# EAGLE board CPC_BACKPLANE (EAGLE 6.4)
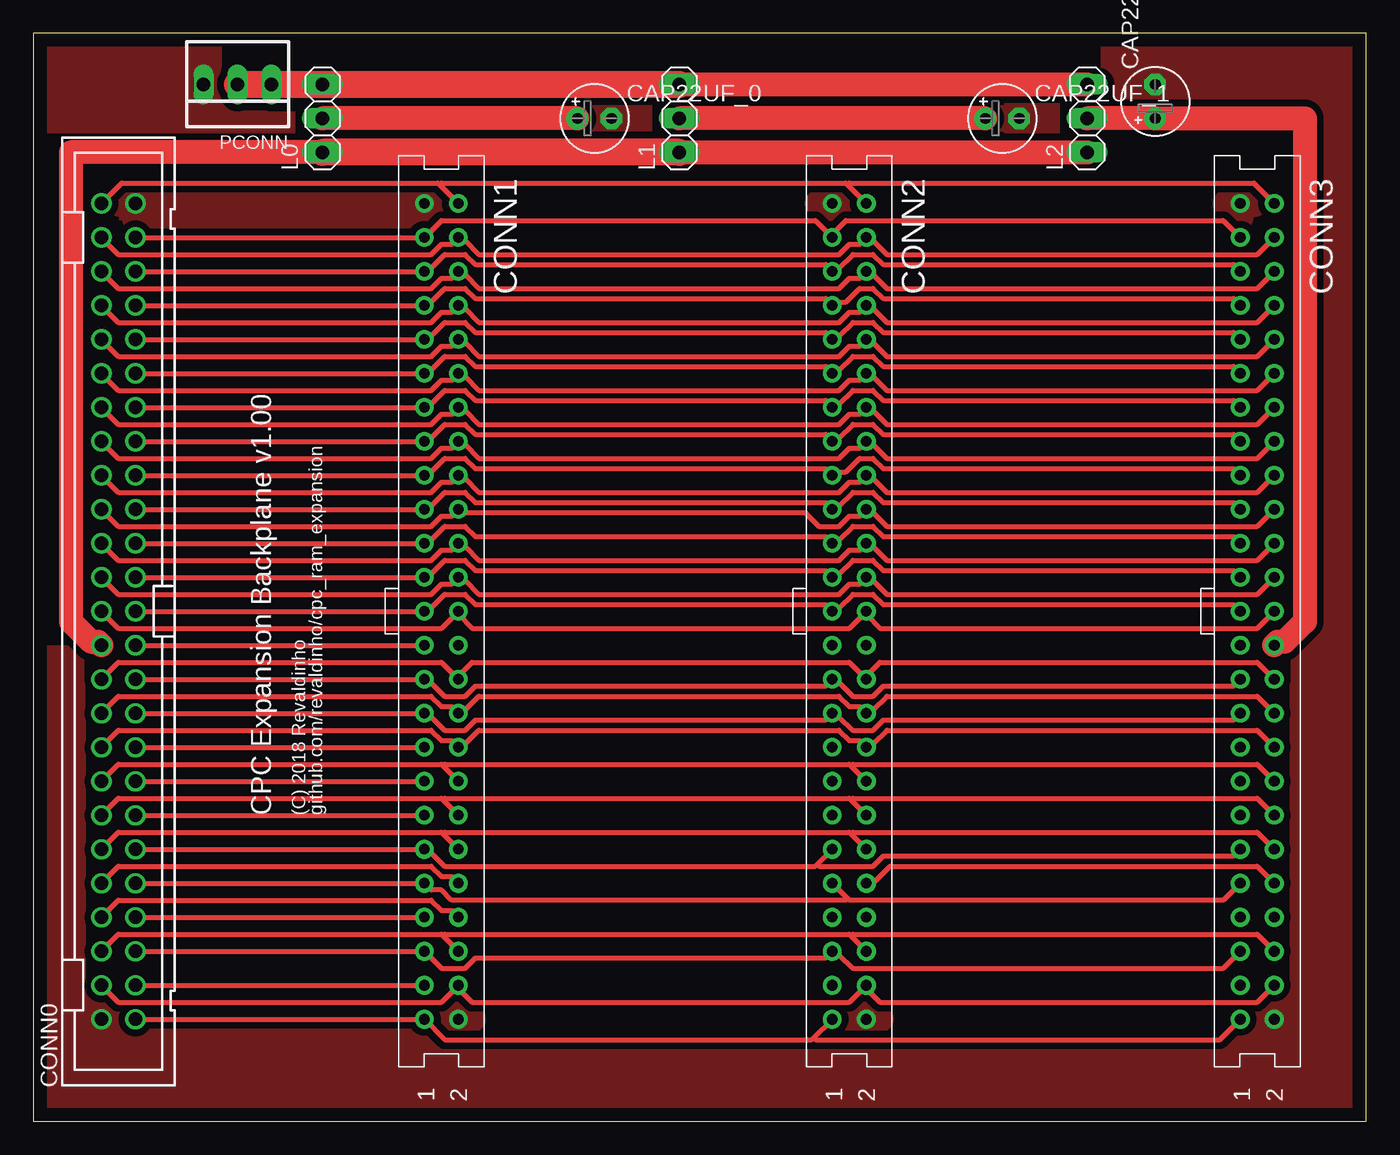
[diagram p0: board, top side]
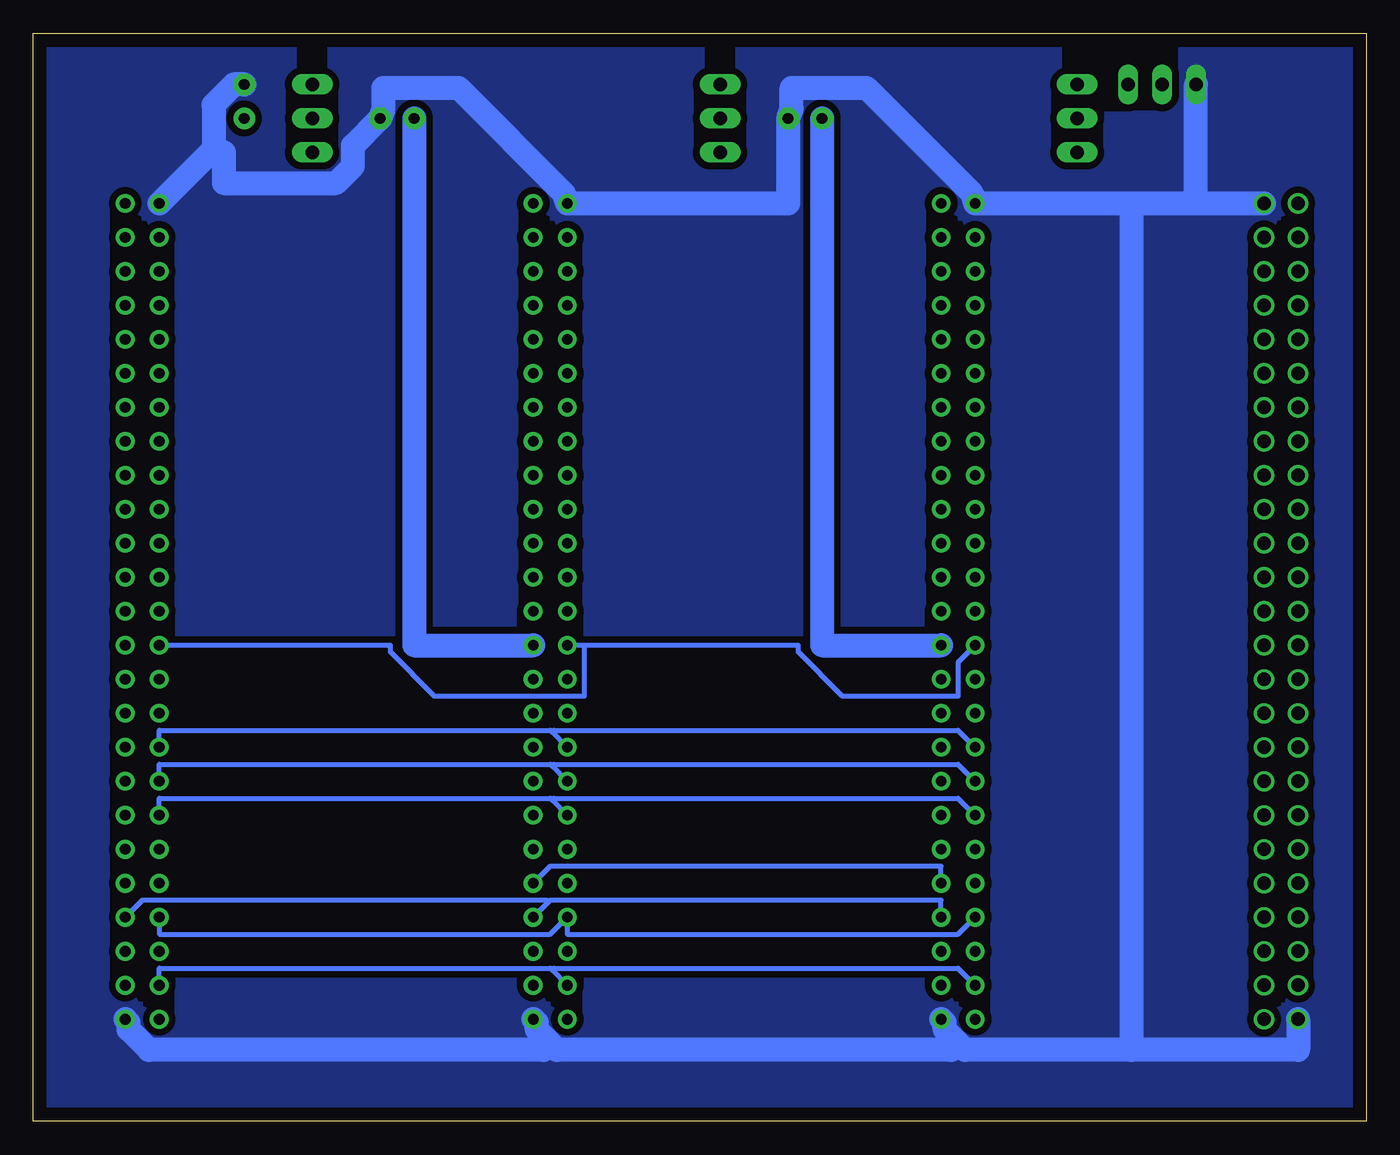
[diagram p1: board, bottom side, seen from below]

Size 99.57 x 81.28 mm. Coordinates in mm from the lower left corner, seen from the top.
Outline: 0,0 99.57,0 99.57,81.28 0,81.28 0,0
Copper layers (1*16): Top 0.035mm / dielectric 1.5mm / Bottom 0.035mm
Design rules "default": minimum track width 10mil, minimum drill 24mil, track to track 8mil, track to pad 8mil, pad to pad 8mil, via to via 8mil, smd to smd 8mil, copper to edge 40mil, drill to drill 8mil, minimum pad ring 10mil, minimum via ring 8mil, stop-mask expansion 4mil, vias tented up to drill 0mil, thermal gap 10mil
Net classes: 0 signal: width 0.381 mm, clearance 0.254 mm; 1 supply: width 1.778 mm, clearance 0.508 mm

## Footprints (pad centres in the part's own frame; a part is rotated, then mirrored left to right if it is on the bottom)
E2,5-5 = drill 0.813 pad 1.6: + -1.27,0 | drill 0.813 pad 1.6 octagon: - 1.27,0
PAK100/2500-50 = drill 1 pad 1.422: 1 -30.48,-1.27; 2 -30.48,1.27; 3 -27.94,-1.27; 4 -27.94,1.27; 5 -25.4,-1.27; 6 -25.4,1.27; 7 -22.86,-1.27; 8 -22.86,1.27; 9 -20.32,-1.27; 10 -20.32,1.27; 11 -17.78,-1.27; 12 -17.78,1.27; 13 -15.24,-1.27; 14 -15.24,1.27; 15 -12.7,-1.27; 16 -12.7,1.27; 17 -10.16,-1.27; 18 -10.16,1.27; 19 -7.62,-1.27; 20 -7.62,1.27; 21 -5.08,-1.27; 22 -5.08,1.27; 23 -2.54,-1.27; 24 -2.54,1.27; 25 0,-1.27; 26 0,1.27; 27 2.54,-1.27; 28 2.54,1.27; 29 5.08,-1.27; 30 5.08,1.27; 31 7.62,-1.27; 32 7.62,1.27; 33 10.16,-1.27; 34 10.16,1.27; 35 12.7,-1.27; 36 12.7,1.27; 37 15.24,-1.27; 38 15.24,1.27; 39 17.78,-1.27; 40 17.78,1.27; 41 20.32,-1.27; 42 20.32,1.27; 43 22.86,-1.27; 44 22.86,1.27; 45 25.4,-1.27; 46 25.4,1.27; 47 27.94,-1.27; 48 27.94,1.27; 49 30.48,-1.27; 50 30.48,1.27
S50V = drill 0.8 pad 1.4: 1 30.48,-1.27; 2 30.48,1.27; 3 27.94,-1.27; 4 27.94,1.27; 5 25.4,-1.27; 6 25.4,1.27; 7 22.86,-1.27; 8 22.86,1.27; 9 20.32,-1.27; 10 20.32,1.27; 11 17.78,-1.27; 12 17.78,1.27; 13 15.24,-1.27; 14 15.24,1.27; 15 12.7,-1.27; 16 12.7,1.27; 17 10.16,-1.27; 18 10.16,1.27; 19 7.62,-1.27; 20 7.62,1.27; 21 5.08,-1.27; 22 5.08,1.27; 23 2.54,-1.27; 24 2.54,1.27; 25 0,-1.27; 26 0,1.27; 27 -2.54,-1.27; 28 -2.54,1.27; 29 -5.08,-1.27; 30 -5.08,1.27; 31 -7.62,-1.27; 32 -7.62,1.27; 33 -10.16,-1.27; 34 -10.16,1.27; 35 -12.7,-1.27; 36 -12.7,1.27; 37 -15.24,-1.27; 38 -15.24,1.27; 39 -17.78,-1.27; 40 -17.78,1.27; 41 -20.32,-1.27; 42 -20.32,1.27; 43 -22.86,-1.27; 44 -22.86,1.27; 45 -25.4,-1.27; 46 -25.4,1.27; 47 -27.94,-1.27; 48 -27.94,1.27; 49 -30.48,-1.27; 50 -30.48,1.27
1X03 = drill 1.016 long: 1 -2.54,0; 2 0,0; 3 2.54,0
22-23-2031 = drill 1 long: 1 -2.54,0; 2 0,0; 3 2.54,0

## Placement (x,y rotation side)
CAP22UF_0  [E2,5-5]  41.91,74.93 0 top
CAP22UF_1  [E2,5-5]  72.39,74.93 0 top
CAP22UF_2  [E2,5-5]  83.82,76.2 90 top
CONN0  [PAK100/2500-50]  6.35,38.1 90 top
CONN1  [S50V]  30.48,38.1 270 top
CONN2  [S50V]  60.96,38.1 270 top
CONN3  [S50V]  91.44,38.1 270 top
L0  [1X03]  21.59,74.93 90 top
L1  [1X03]  48.26,74.93 90 top
L2  [1X03]  78.74,74.93 90 top
PCONN  [22-23-2031]  15.24,77.47 180 top

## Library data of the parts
CAP22UF_0 CAP22UF_1 CAP22UF_2 = resistor
CONN0 = con-3m
CONN1-CONN3 = con-3m-skt-header
L0 L1 L2 = pinhead
PCONN = con-molex

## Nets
A0: CONN0.33 CONN1.33 CONN2.33 CONN3.33
A1: CONN0.34 CONN1.34 CONN2.34 CONN3.34
A2: CONN0.35 CONN1.35 CONN2.35 CONN3.35
A3: CONN0.36 CONN1.36 CONN2.36 CONN3.36
A4: CONN0.37 CONN1.37 CONN2.37 CONN3.37
A5: CONN0.38 CONN1.38 CONN2.38 CONN3.38
A6: CONN0.39 CONN1.39 CONN2.39 CONN3.39
A7: CONN0.40 CONN1.40 CONN2.40 CONN3.40
A8: CONN0.41 CONN1.41 CONN2.41 CONN3.41
A9: CONN0.42 CONN1.42 CONN2.42 CONN3.42
A10: CONN0.43 CONN1.43 CONN2.43 CONN3.43
A11: CONN0.44 CONN1.44 CONN2.44 CONN3.44
A12: CONN0.45 CONN1.45 CONN2.45 CONN3.45
A13: CONN0.46 CONN1.46 CONN2.46 CONN3.46
A14: CONN0.47 CONN1.47 CONN2.47 CONN3.47
A15: CONN0.48 CONN1.48 CONN2.48 CONN3.48
BUSACK_B: CONN0.13 CONN1.13 CONN2.13 CONN3.13
BUSRESET_B: CONN0.11 CONN1.11 CONN2.11 CONN3.11
BUSRQ_B: CONN0.14 CONN1.14 CONN2.14 CONN3.14
CLK: CONN0.1 CONN1.1 CONN2.1 CONN3.1
CURSOR: CONN0.5 CONN1.5 CONN2.5 CONN3.5
D0: CONN0.25 CONN1.25 CONN2.25 CONN3.25
D1: CONN0.26 CONN1.26 CONN2.26 CONN3.26
D2: CONN0.27 CONN1.27 CONN2.27 CONN3.27
D3: CONN0.28 CONN1.28 CONN2.28 CONN3.28
D4: CONN0.29 CONN1.29 CONN2.29 CONN3.29
D5: CONN0.30 CONN1.30 CONN2.30 CONN3.30
D6: CONN0.31 CONN1.31 CONN2.31 CONN3.31
D7: CONN0.32 CONN1.32 CONN2.32 CONN3.32
EXP_B: CONN0.3 CONN1.3 CONN2.3 CONN3.3
HALT_B: CONN0.17 CONN1.17 CONN2.17 CONN3.17
INT_B: CONN0.16 CONN1.16 CONN2.16 CONN3.16
IOREQ_B: CONN0.20 CONN1.20 CONN2.20 CONN3.20
LPEN: CONN0.4 CONN1.4 CONN2.4 CONN3.4
M1_B: CONN0.22 CONN1.22 CONN2.22 CONN3.22
MREQ_B: CONN0.23 CONN1.23 CONN2.23 CONN3.23
NMI_B: CONN0.15 CONN1.15 CONN2.15 CONN3.15
RAMDIS: CONN0.6 CONN1.6 CONN2.6 CONN3.6
RAMRD_B: CONN0.7 CONN1.7 CONN2.7 CONN3.7
RD_B: CONN0.19 CONN1.19 CONN2.19 CONN3.19
READY: CONN0.12 CONN1.12 CONN2.12 CONN3.12
RESET_B: CONN0.10 CONN1.10 CONN2.10 CONN3.10
RFSH_B: CONN0.21 CONN1.21 CONN2.21 CONN3.21
ROMDIS: CONN0.8 CONN1.8 CONN2.8 CONN3.8
ROMEN_B: CONN0.9 CONN1.9 CONN2.9 CONN3.9
SOUND: CONN0.50 CONN1.50 CONN2.50 CONN3.50
VDD [supply]: CAP22UF_0.+ CONN1.24 L0.2
VDD2 [supply]: CAP22UF_1.+ CONN2.24 L1.2
VDD3 [supply]: CAP22UF_2.+ CONN3.24 L2.2
VDD_CPC [supply]: CONN0.24 L0.1 L1.1 L2.1
VDD_EXT [supply]: L0.3 L1.3 L2.3 PCONN.1 PCONN.2
VSS [supply]: CAP22UF_0.- CAP22UF_1.- CAP22UF_2.- CONN0.2 CONN0.49 CONN1.2 CONN1.49 CONN2.2 CONN2.49 CONN3.2 CONN3.49 PCONN.3
WR_B: CONN0.18 CONN1.18 CONN2.18 CONN3.18

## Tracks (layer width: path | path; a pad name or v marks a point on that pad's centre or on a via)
A0
  Top 0.381: CONN0.33 CONN1.33 29.46,48.26 30.73,49.53 32.26,49.53 33.02,48.77 59.18,48.77 CONN2.33 59.69,48.51 60.71,48.51 61.72,49.53 62.74,49.53 63.5,48.77 89.66,48.77 CONN3.33
A1
  Top 0.381: CONN0.34 6.35,46.99 29.72,46.99 30.48,47.75 31.24,47.75 CONN1.34 31.75,48.01 32.26,48.01 33.27,46.99 60.2,46.99 60.96,47.75 61.72,47.75 CONN2.34 62.23,48.01 62.74,48.01 63.75,46.99 91.44,46.99 CONN3.34
A2
  Top 0.381: CONN0.35 CONN1.35 29.46,50.8 30.73,52.07 32.26,52.07 33.02,51.31 59.18,51.31 CONN2.35 59.69,51.05 60.2,51.05 61.21,52.07 62.74,52.07 63.5,51.31 89.66,51.31 CONN3.35
A3
  Top 0.381: CONN0.36 6.35,49.53 29.72,49.53 30.48,50.29 31.24,50.29 CONN1.36 31.75,50.55 32.26,50.55 33.27,49.53 60.2,49.53 60.96,50.29 61.72,50.29 CONN2.36 62.23,50.55 62.74,50.55 63.75,49.53 91.44,49.53 CONN3.36
A4
  Top 0.381: CONN0.37 CONN1.37 29.46,53.34 30.73,54.61 32.26,54.61 33.02,53.85 59.18,53.85 CONN2.37 59.69,53.59 60.2,53.59 61.21,54.61 62.74,54.61 63.5,53.85 89.66,53.85 CONN3.37
A5
  Top 0.381: CONN0.38 6.35,52.07 29.72,52.07 30.48,52.83 31.24,52.83 CONN1.38 31.75,53.09 32.26,53.09 33.27,52.07 60.2,52.07 60.96,52.83 61.72,52.83 CONN2.38 62.23,53.09 62.74,53.09 63.75,52.07 91.44,52.07 CONN3.38
A6
  Top 0.381: CONN0.39 CONN1.39 29.46,55.88 30.73,57.15 32.26,57.15 33.02,56.39 59.18,56.39 CONN2.39 59.69,56.13 60.2,56.13 61.21,57.15 62.74,57.15 63.5,56.39 89.66,56.39 CONN3.39
A7
  Top 0.381: CONN0.40 6.35,54.61 29.72,54.61 30.48,55.37 31.24,55.37 CONN1.40 31.75,55.63 32.26,55.63 33.27,54.61 60.2,54.61 60.96,55.37 61.72,55.37 CONN2.40 62.23,55.63 62.74,55.63 63.75,54.61 91.44,54.61 CONN3.40
A8
  Top 0.381: CONN0.41 CONN1.41 29.46,58.42 30.73,59.69 32.26,59.69 33.02,58.93 59.18,58.93 CONN2.41 59.69,58.67 60.2,58.67 61.21,59.69 62.74,59.69 63.5,58.93 89.66,58.93 CONN3.41
A9
  Top 0.381: CONN0.42 6.35,57.15 29.72,57.15 30.48,57.91 31.24,57.91 CONN1.42 31.75,58.17 32.26,58.17 33.27,57.15 60.2,57.15 60.96,57.91 61.72,57.91 CONN2.42 62.23,58.17 62.74,58.17 63.75,57.15 91.44,57.15 CONN3.42
A10
  Top 0.381: CONN0.43 CONN1.43 29.46,60.96 30.73,62.23 32.26,62.23 33.02,61.47 59.18,61.47 CONN2.43 59.69,61.21 60.71,61.21 61.72,62.23 62.74,62.23 63.5,61.47 89.66,61.47 CONN3.43
A11
  Top 0.381: CONN0.44 6.35,59.69 29.72,59.69 30.48,60.45 31.24,60.45 CONN1.44 31.75,60.71 32.26,60.71 33.27,59.69 60.2,59.69 60.96,60.45 61.72,60.45 CONN2.44 62.23,60.71 62.74,60.71 63.75,59.69 91.44,59.69 CONN3.44
A12
  Top 0.381: CONN0.45 CONN1.45 29.46,63.5 30.73,64.77 32.26,64.77 33.02,64.01 59.18,64.01 CONN2.45 59.69,63.75 60.2,63.75 61.21,64.77 62.74,64.77 63.5,64.01 89.66,64.01 CONN3.45
A13
  Top 0.381: CONN0.46 6.35,62.23 29.72,62.23 30.48,62.99 31.24,62.99 CONN1.46 31.75,63.25 32.26,63.25 33.27,62.23 60.2,62.23 60.96,62.99 61.72,62.99 CONN2.46 62.23,63.25 62.74,63.25 63.75,62.23 91.44,62.23 CONN3.46
A14
  Top 0.381: CONN0.47 CONN1.47 30.48,67.31 58.42,67.31 CONN2.47 59.69,66.29 60.71,67.31 88.9,67.31 CONN3.47
A15
  Top 0.381: CONN0.48 6.35,64.77 29.72,64.77 30.48,65.53 31.24,65.53 CONN1.48 31.75,65.79 32.26,65.79 33.27,64.77 60.2,64.77 60.96,65.53 61.72,65.53 CONN2.48 62.23,65.79 62.74,65.79 63.75,64.77 91.44,64.77 CONN3.48
BUSACK_B
  Top 0.381: CONN0.13 CONN1.13
  Bottom 0.381: 60.83,24 60.96,24.13 90.17,24.13 CONN3.13 | 60.83,24 CONN2.13 | CONN1.13 30.48,24.13 60.71,24.13 60.83,24
BUSRESET_B
  Top 0.381: CONN0.11 CONN1.11 29.46,20.32 30.73,19.05 58.42,19.05 58.55,19.18 | 58.55,19.18 CONN2.11 | CONN3.11 89.66,19.81 63.5,19.81 62.74,19.05 58.67,19.05 58.55,19.18
BUSRQ_B
  Top 0.381: 30.61,24 30.48,24.13 6.35,24.13 CONN0.14 | 30.61,24 CONN1.14 | 61.09,24 60.96,24.13 30.73,24.13 30.61,24 | 61.09,24 CONN2.14 | CONN3.14 91.44,24.13 61.21,24.13 61.09,24
CLK
  Top 0.381: CONN0.1 CONN1.1 30.73,6.1 58.17,6.1 58.29,6.22 | 58.29,6.22 CONN2.1 | CONN3.1 88.65,6.1 58.42,6.1 58.29,6.22
CURSOR
  Top 0.381: CONN0.5 CONN1.5 30.48,11.43 32.26,11.43 33.02,12.19 59.18,12.19 CONN2.5 59.69,12.45 60.2,12.45 61.21,11.43 88.9,11.43 CONN3.5
D0
  Top 0.381: CONN0.25 CONN1.25 29.46,38.1 30.73,39.37 32.26,39.37 33.02,38.61 59.18,38.61 CONN2.25 59.69,38.35 60.2,38.35 61.21,39.37 62.74,39.37 63.5,38.61 89.66,38.61 CONN3.25
D1
  Top 0.381: CONN0.26 6.35,36.83 30.48,36.83 CONN1.26 31.75,37.85 32.77,36.83 60.96,36.83 CONN2.26 62.23,37.85 63.25,36.83 91.44,36.83 CONN3.26
D2
  Top 0.381: CONN0.27 CONN1.27 29.46,40.64 30.73,41.91 32.26,41.91 33.02,41.15 59.18,41.15 CONN2.27 59.69,40.89 60.2,40.89 61.21,41.91 62.74,41.91 63.5,41.15 89.66,41.15 CONN3.27
D3
  Top 0.381: CONN0.28 6.35,39.37 29.72,39.37 30.48,40.13 31.24,40.13 CONN1.28 31.75,40.39 32.26,40.39 33.27,39.37 60.2,39.37 60.96,40.13 61.72,40.13 CONN2.28 62.23,40.39 62.74,40.39 63.75,39.37 91.44,39.37 CONN3.28
D4
  Top 0.381: CONN0.29 CONN1.29 29.46,43.18 30.73,44.45 32.26,44.45 33.02,43.69 59.18,43.69 CONN2.29 59.69,43.43 60.2,43.43 61.21,44.45 62.74,44.45 63.5,43.69 89.66,43.69 CONN3.29
D5
  Top 0.381: CONN0.30 6.35,41.91 29.72,41.91 30.48,42.67 31.24,42.67 CONN1.30 31.75,42.93 32.26,42.93 33.27,41.91 60.2,41.91 60.96,42.67 61.72,42.67 CONN2.30 62.23,42.93 62.74,42.93 63.75,41.91 91.44,41.91 CONN3.30
D6
  Top 0.381: CONN0.31 CONN1.31 29.46,45.72 30.73,46.99 32.26,46.99 33.02,46.23 59.18,46.23 CONN2.31 59.69,45.97 60.2,45.97 61.21,46.99 62.74,46.99 63.5,46.23 89.66,46.23 CONN3.31
D7
  Top 0.381: CONN0.32 6.35,44.45 29.72,44.45 30.48,45.21 31.24,45.21 CONN1.32 31.75,45.47 57.66,45.47 58.67,44.45 60.2,44.45 60.96,45.21 61.72,45.21 CONN2.32 62.23,45.47 62.74,45.47 63.75,44.45 91.44,44.45 CONN3.32
EXP_B
  Top 0.381: CONN0.3 CONN1.3
  Bottom 0.381: 60.83,11.3 60.96,11.43 90.17,11.43 CONN3.3 | 60.83,11.3 CONN2.3 | CONN1.3 30.48,11.43 60.71,11.43 60.83,11.3
HALT_B
  Top 0.381: CONN0.17 CONN1.17
  Bottom 0.381: 60.83,29.08 60.96,29.21 90.17,29.21 CONN3.17 | 60.83,29.08 CONN2.17 | CONN1.17 30.48,29.21 60.71,29.21 60.83,29.08
INT_B
  Top 0.381: 30.61,26.54 30.48,26.67 6.35,26.67 CONN0.16 | 30.61,26.54 CONN1.16 | 61.09,26.54 60.96,26.67 30.73,26.67 30.61,26.54 | 61.09,26.54 CONN2.16 | CONN3.16 91.44,26.67 61.21,26.67 61.09,26.54
IOREQ_B
  Top 0.381: CONN0.20 6.35,31.75 29.72,31.75 30.48,30.99 31.24,30.99 CONN1.20 31.75,30.73 32.26,30.73 33.27,31.75 60.2,31.75 60.96,30.99 61.72,30.99 CONN2.20 62.23,30.73 62.74,30.73 63.75,31.75 91.44,31.75 CONN3.20
LPEN
  Top 0.381: CONN0.4 6.35,8.89 30.48,8.89 CONN1.4 31.75,9.91 32.77,8.89 60.96,8.89 CONN2.4 62.23,9.91 63.25,8.89 91.44,8.89 CONN3.4
M1_B
  Top 0.381: CONN0.22 6.35,34.29 30.48,34.29 CONN1.22 31.75,33.27 32.77,34.29 60.96,34.29 CONN2.22 62.23,33.27 63.25,34.29 91.44,34.29 CONN3.22
MREQ_B
  Top 0.381: CONN0.23 CONN1.23
  Bottom 0.381: 58.42,35.56 42.42,35.56 42.42,35.05 39.12,31.75 30.48,31.75 30.48,34.29 CONN1.23 | 58.42,35.56 CONN2.23 | CONN3.23 72.9,35.56 72.9,35.05 69.6,31.75 58.42,31.75 58.42,35.56
NMI_B
  Top 0.381: CONN0.15 CONN1.15
  Bottom 0.381: 60.83,26.54 60.96,26.67 90.17,26.67 CONN3.15 | 60.83,26.54 CONN2.15 | CONN1.15 30.48,26.67 60.71,26.67 60.83,26.54
RAMDIS
  Top 0.381: 30.61,13.84 30.48,13.97 6.35,13.97 CONN0.6 | 30.61,13.84 CONN1.6 | 61.09,13.84 60.96,13.97 30.73,13.97 30.61,13.84 | 61.09,13.84 CONN2.6 | CONN3.6 91.44,13.97 61.21,13.97 61.09,13.84
RAMRD_B
  Top 0.381: CONN0.7 CONN1.7
  Bottom 0.381: CONN3.7 90.17,13.97 60.96,13.97 CONN2.7 59.69,13.97 30.48,13.97 CONN1.7
RD_B
  Top 0.381: CONN0.19 CONN1.19 29.46,30.48 30.73,29.21 32.26,29.21 33.02,29.97 59.18,29.97 CONN2.19 59.69,30.23 60.2,30.23 61.21,29.21 62.74,29.21 63.5,29.97 89.66,29.97 CONN3.19
READY
  Top 0.381: 30.61,21.46 30.48,21.59 6.35,21.59 CONN0.12 | 30.61,21.46 CONN1.12 | 61.09,21.46 60.96,21.59 30.73,21.59 30.61,21.46 | 61.09,21.46 CONN2.12 | CONN3.12 91.44,21.59 61.21,21.59 61.09,21.46
RESET_B
  Top 0.381: CONN1.10 31.24,18.29 30.48,18.29 29.72,19.05 6.35,19.05 CONN0.10 | CONN3.10 91.44,19.05 64.01,19.05 62.74,17.78 CONN2.10
  Bottom 0.381: CONN2.10 60.96,19.05 31.75,19.05 CONN1.10
RFSH_B
  Top 0.381: CONN0.21 CONN1.21 29.46,33.02 30.73,31.75 32.26,31.75 33.02,32.51 59.18,32.51 CONN2.21 59.69,32.77 60.2,32.77 61.21,31.75 62.74,31.75 63.5,32.51 89.66,32.51 CONN3.21
ROMDIS
  Top 0.381: CONN1.8 31.24,15.75 30.48,15.75 29.72,16.51 6.35,16.51 CONN0.8
  Bottom 0.381: 61.09,16.38 60.96,16.51 31.75,16.51 CONN1.8 | 61.09,16.38 CONN2.8 | CONN3.8 91.44,16.51 61.21,16.51 61.09,16.38
ROMEN_B
  Top 0.381: CONN0.9 CONN1.9 29.72,17.27 30.48,17.27 31.24,16.51 60.71,16.51 60.83,16.64 | 60.83,16.64 60.96,16.51 88.9,16.51 CONN3.9 | 60.83,16.64 CONN2.9
SOUND
  Top 0.381: 30.35,69.98 30.23,70.1 6.6,70.1 CONN0.50 | 30.35,69.98 CONN1.50 | 60.83,69.98 60.71,70.1 30.48,70.1 30.35,69.98 | 60.83,69.98 CONN2.50 | CONN3.50 91.19,70.1 60.96,70.1 60.83,69.98
VDD
  Top 1.778: CAP22UF_0.+ L0.2
  Bottom 1.778: CONN1.24 40.64,35.56 CAP22UF_0.+
VDD2
  Top 1.778: CAP22UF_1.+ L1.2
  Bottom 1.778: CONN2.24 71.12,35.56 CAP22UF_1.+
VDD3
  Top 1.778: CONN3.24 92.96,35.81 93.47,35.81 95,37.34 95,74.93 CAP22UF_2.+ L2.2
VDD_CPC
  Top 1.778: L1.1 L2.1 | CONN0.24 4.83,35.81 4.32,35.81 2.79,37.34 2.79,72.39 L0.1
  Top 2.032: L1.1 L0.1
VDD_EXT
  Top 1.778: L1.3 L2.3
  Top 2.032: PCONN.2 PCONN.1 L0.3 L1.3
VSS
  Bottom 1.778: CONN1.2 31.5,7.37 31.5,6.86 30.48,5.84 | 30.48,5.84 29.97,5.33 17.53,5.33 | 17.53,5.33 5.08,5.33 CONN0.2 | CONN2.2 61.98,7.37 61.98,6.86 60.96,5.84 | 60.96,5.84 60.45,5.33 30.99,5.33 30.48,5.84 | CONN3.2 92.46,7.37 92.46,6.86 90.93,5.33 61.47,5.33 60.96,5.84 | CONN0.49 12.7,68.58 | 12.7,68.58 17.53,68.58 | 17.53,68.58 CONN1.49 29.46,69.34 37.34,77.22 42.93,77.22 42.93,75.69 CAP22UF_0.- 43.18,68.58 CONN2.49 59.94,69.34 67.82,77.22 73.41,77.22 73.41,75.69 CAP22UF_1.- 75.69,72.9 75.69,71.37 76.96,70.1 85.34,70.1 85.34,72.39 86.11,72.64 | 12.7,68.58 PCONN.3 | 86.11,72.64 CONN3.49 | 86.11,72.64 86.11,75.95 84.58,77.47 CAP22UF_2.- | 17.53,68.58 17.53,5.33
  pour Top: 0,0 0,81.28 99.57,81.28 100.33,81.28 100.33,0
  pour Bottom: 0,0 0,81.28 99.57,81.28 100.33,81.28 100.33,0
WR_B
  Top 0.381: CONN0.18 6.35,29.21 29.72,29.21 30.48,28.45 31.24,28.45 CONN1.18 31.75,28.19 32.26,28.19 33.27,29.21 60.2,29.21 60.96,28.45 61.72,28.45 CONN2.18 62.23,28.19 62.74,28.19 63.75,29.21 91.44,29.21 CONN3.18

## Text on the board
tPlace: CPC Expansion Backplane v1.00 | (C) 2018 Revaldinho | github.com/revaldinho/cpc_ram_expansion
